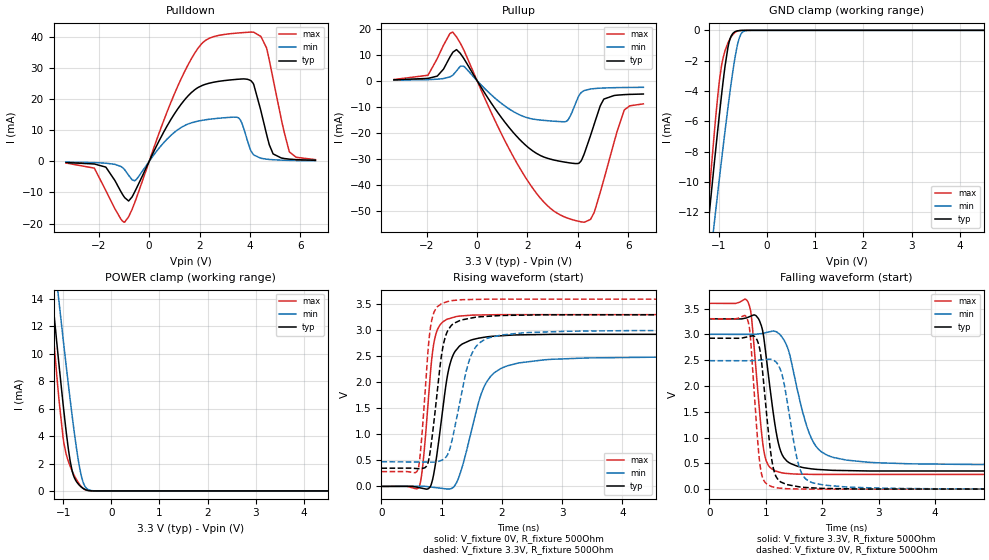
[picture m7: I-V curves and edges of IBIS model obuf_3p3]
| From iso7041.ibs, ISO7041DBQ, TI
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|   obuf_3p3 Model
[Model]   obuf_3p3
Model_type   3-state
Polarity   Non-Inverting
Vmeas = 1.65
Vref = 0
Cref = 2pF
Rref = 100000
|   typ   min   max
C_comp   0.461pF   0.430pF   0.522pF
| Where Nom  PVT is Nominal Process, 3.3V, 27C
|   Fast PVT is Strong Process,  3.6V, -55C
|   Slow PVT is Weak Process,   3.0V, 150C
[Voltage Range]   3.3   3   3.6
|Junction Temperature
[Temperature Range]   27   150   -55
[Pullup Reference]   3.3   3   3.6
[Pulldown Reference]   0   0   0
[Power Clamp Reference]   3.3   3   3.6
[GND Clamp Reference]   0   0   0
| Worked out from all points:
|   slope of the pulldown table from 0 to 0.495 V, typ, clamps not added: 60.5 ohm
|   slope of the pullup table from 0 to 0.495 V, typ, clamps not added: 64.9 ohm
|   GND clamp passes 1 mA (typ) near -0.81 V on its own axis
|   POWER clamp passes 1 mA (typ) near -0.77 V on its own axis
|   falling waveform, V_fixture 3.3V, R_fixture 500Ohm: 20-80 % time 223ps typ, 363ps min, 161ps max; typ from 3.3 V to 0.349 V
|   rising waveform, V_fixture 0V, R_fixture 500Ohm: 20-80 % time 218ps typ, 368ps min, 148ps max; typ from 0 V to 2.92 V
|   rising waveform, V_fixture 3.3V, R_fixture 500Ohm: 20-80 % time 186ps typ, 292ps min, 131ps max; typ from 0.349 V to 3.3 V
|   falling waveform, V_fixture 0V, R_fixture 500Ohm: 20-80 % time 166ps typ, 242ps min, 130ps max; typ from 2.92 V to 0 V
[Pulldown]
|   Voltage   I(typ)   I(min)   I(max)
-3.3V     -363.2uA   -210.5uA   -522.9uA
-2.171V   -837.9uA   -383.6uA   -2.229mA
-973.5mV  -11.65mA   -2.651mA   -19.58mA
-547.8mV  -9.398mA   -6.103mA   -12.72mA
848.1mV   13.3mA     8.268mA    18.73mA
1.888V    23.53mA    12.88mA    35.85mA
3.551V    26.47mA    14.01mA    41.38mA
4.046V    25.95mA    3.305mA    41.65mA
4.66V     8.762mA    721uA      36.54mA
4.917V    2.48mA     539.2uA    26.65mA
5.57V     725.7uA    327.8uA    3.014mA
6.6V      352uA      202.1uA    566.6uA
[GND Clamp]
|   Voltage   I(typ)   I(min)   I(max)
-3.3V     -83.3mA    -77.84mA   -98.23mA
-1.36V    -17.26mA   -20.19mA   -16.99mA
-1.221V   -12.72mA   -16.21mA   -11.47mA
-1.102V   -8.932mA   -12.84mA   -6.951mA
-1.003V   -5.897mA   -10.1mA    -3.662mA
-943.8mV  -4.179mA   -8.482mA   -2.275mA
-874.5mV  -2.37mA    -6.644mA   -1.352mA
-795.3mV  -852.9uA   -4.636mA   -703.8uA
-646.8mV  -64.87uA   -1.436mA   -97.67uA
-547.8mV  -8.624uA   -277.9uA   -10.36uA
-399.3mV  -218.6nA   -6.815uA   -104.2nA
6.6V      0A         0A         0A
[Pullup]
|   Voltage   I(typ)   I(min)   I(max)
-3.3V     309.9uA    180.5uA    428.1uA
-1.944V   876.5uA    388.7uA    2.14mA
-953.7mV  11mA       2.186mA    18.57mA
-537.9mV  8.705mA    5.601mA    12.03mA
986.7mV   -14.47mA   -8.917mA   -20.86mA
2.095V    -26.22mA   -14.54mA   -39.82mA
3.551V    -31.47mA   -15.63mA   -52.77mA
4.234V    -28.65mA   -3.913mA   -54.49mA
4.64V     -17.05mA   -3.061mA   -50.93mA
5.026V    -7.175mA   -2.823mA   -38.28mA
5.838V    -5.383mA   -2.637mA   -11.46mA
6.6V      -5.149mA   -2.569mA   -8.933mA
[POWER Clamp]
|   Voltage   I(typ)   I(min)   I(max)
-3.3V     93.73mA    88.82mA    106.4mA
-1.33V    18.02mA    21.73mA    16.76mA
-1.221V   14.02mA    18.16mA    12.08mA
-1.102V   9.767mA    14.31mA    7.251mA
-983.4mV  5.753mA    10.56mA    3.469mA
-884.4mV  2.872mA    7.543mA    2.083mA
-815.1mV  1.489mA    5.536mA    1.468mA
-656.7mV  393.5uA    1.671mA    464.2uA
-587.4mV  188.4uA    655.2uA    193.6uA
-528mV    79.48uA    237.5uA    64.26uA
-260.7mV  84.93nA    1.053uA    159.2nA
6.6V      0A         0A         0A
[Ramp]
R_load = 500
|   typ   min   max
dV/dt_r   1.75494/2.18004e-10   1.49367/3.67906e-10   1.98142/1.47631e-10
dV/dt_f   1.77031/2.22559e-10   1.51603/3.63362e-10   1.98971/1.6107e-10
[Falling Waveform]
V_fixture = 3.3V
V_fixture_min = 3V
V_fixture_max = 3.6V
R_fixture = 500Ohm
C_fixture = 0F
|   Time   V(typ)   V(min)   V(max)
0s        3.3V       3V         3.6V
686.3ps   3.331V     2.999V     3.622V
743.8ps   3.356V     2.999V     3.36V
868.7ps   3.306V     3.008V     1.775V
1.011ns   2.533V     3.035V     540.1mV
1.242ns   812.5mV    3.006V     329.7mV
1.502ns   469.6mV    2.216V     293.5mV
1.986ns   377.8mV    723.2mV    285.6mV
3.579ns   352.1mV    490.5mV    285.6mV
100ns     349.5mV    473.3mV    283.8mV
[Rising Waveform]
V_fixture = 0V
V_fixture_min = 0V
V_fixture_max = 0V
R_fixture = 500Ohm
C_fixture = 0F
|   Time   V(typ)   V(min)   V(max)
0s        -321.1nV   4.686nV    -272.9pV
632ps     -25.48mV   1.217mV    7.794mV
807.1ps   -11.99mV   -10.46mV   2.092V
916.4ps   582.1mV    -25.84mV   2.974V
1.136ns   2.344V     -47.16mV   3.228V
1.502ns   2.817V     1.112V     3.292V
1.713ns   2.868V     1.939V     3.296V
1.986ns   2.895V     2.268V     3.301V
3.415ns   2.922V     2.468V     3.301V
100ns     2.925V     2.489V     3.302V
[Rising Waveform]
V_fixture = 3.3V
V_fixture_min = 3V
V_fixture_max = 3.6V
R_fixture = 500Ohm
C_fixture = 0F
|   Time   V(typ)   V(min)   V(max)
0s        349.5mV    473.3mV    283.8mV
606.3ps   341.4mV    468.7mV    327mV
761.9ps   419.2mV    467.5mV    2.437V
848ps     1.017V     466.8mV    3.26V
1.034ns   2.757V     524.4mV    3.529V
1.331ns   3.199V     1.792V     3.588V
1.484ns   3.234V     2.505V     3.591V
1.713ns   3.265V     2.824V     3.597V
3.11ns    3.297V     2.982V     3.598V
100ns     3.3V       3V         3.6V
[Falling Waveform]
|Gnd
V_fixture = 0V
V_fixture_min = 0V
V_fixture_max = 0V
R_fixture = 500Ohm
C_fixture = 0F
|   Time   V(typ)   V(min)   V(max)
0s        2.925V     2.489V     3.302V
654.9ps   2.946V     2.488V     3.34V
720.5ps   2.961V     2.488V     3.028V
826.5ps   2.929V     2.496V     1.381V
933.6ps   2.384V     2.505V     255.8mV
1.136ns   398.2mV    2.502V     39.88mV
1.382ns   86.91mV    1.682V     7.562mV
1.713ns   32.38mV    192.5mV    1.614mV
3.11ns    2.79mV     17.89mV    963.8uV
100ns     -321.3nV   776.6pV    -308.2pV
